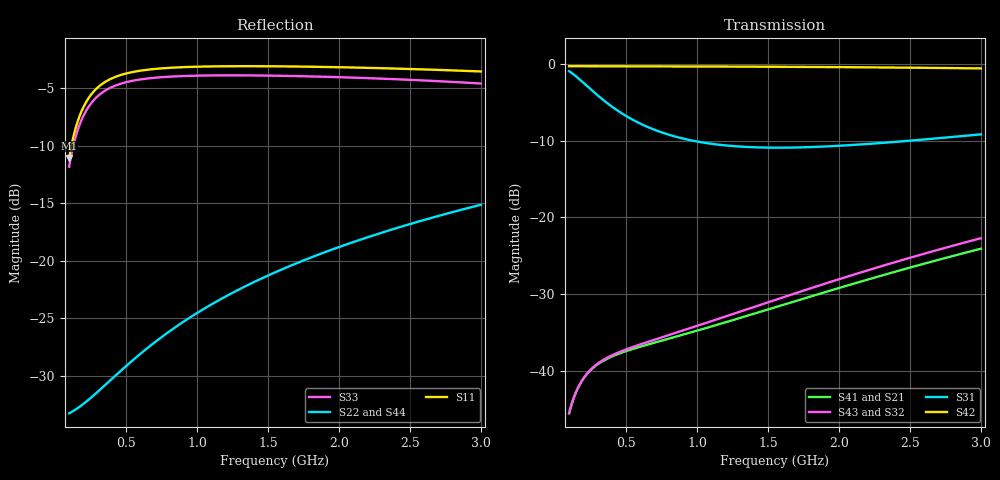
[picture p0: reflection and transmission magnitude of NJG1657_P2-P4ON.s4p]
! NJG1657MD7(1bit control high power DPDT switch) S-parameter
! VDD=2.85V, VCTL(H)=2.6V, VCTL(L)=0V
! P2-P4 ON mode
! Port1...P1, Port2...P2, Port3...P3, Port4...P4
# hz S ma R 50
! 4 Port Network Data from SP1.SP block
! freq  magS11  angS11  magS12  angS12  magS13  angS13  magS14  angS14
!  magS21  angS21  magS22  angS22  magS23  angS23  magS24  angS24
!  magS31  angS31  magS32  angS32  magS33  angS33  magS34  angS34
!  magS41  angS41  magS42  angS42  magS43  angS43  magS44  angS44
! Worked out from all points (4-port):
!   291 points, 100 MHz to 3 GHz, reference 50 ohm
!   strongest paths, dB at 100 MHz, 820 MHz, 1.55 GHz, 2.28 GHz, 3 GHz:
!     S42: -0.2, -0.3, -0.3, -0.4, -0.5
!     S31: -0.9, -9.3, -10.9, -10.3, -9.1
!     S43: -45.6, -35.3, -30.8, -26.5, -22.7
!     S32: -45.6, -35.3, -30.8, -26.5, -22.7
!     S41: -45.6, -35.7, -31.7, -27.7, -24.1
!     S21: -45.6, -35.8, -31.7, -27.7, -24.0
!   lowest |S11| = -11.1 dB at 100 MHz (marker M1), VSWR 1.77, Z = 36.3 - j20.7 ohm
!   |S11| at or under -10 dB: start of sweep to 116.5 MHz
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1e8  0.2791 -110.0  0.005241 66.2  0.9018 -17.0  0.005258 66.2
     0.005241 66.2  0.02173 -15.7  0.005264 67.1  0.9724 -1.3
     0.9018 -17.0  0.005264 67.1  0.256 -109.7  0.005272 67.0
     0.005258 66.2  0.9724 -1.3  0.005272 67.0  0.02178 -15.3
1.7e8  0.4185 -125.0  0.007918 59.8  0.8026 -25.7  0.007943 59.7
       0.007918 59.8  0.02311 -25.6  0.007969 61.2  0.9721 -2.3
       0.8026 -25.7  0.007969 61.2  0.3838 -125.0  0.007981 61.1
       0.007943 59.7  0.9721 -2.3  0.007981 61.1  0.02305 -25.2
2.8e8  0.5488 -141.3  0.01058 52.8  0.6515 -33.7  0.01061 52.7
       0.01058 52.8  0.02623 -38.9  0.0107 55.1  0.9717 -3.7
       0.6515 -33.7  0.0107 55.1  0.5031 -141.4  0.01072 54.9
       0.01061 52.7  0.9717 -3.7  0.01072 54.9  0.02594 -38.5
4.6e8  0.6394 -156.9  0.01295 49.5  0.4857 -37.0  0.01299 49.4
       0.01295 49.5  0.03309 -54.9  0.01326 53.1  0.9711 -6.1
       0.4857 -37.0  0.01326 53.1  0.586 -157.2  0.01328 52.8
       0.01299 49.4  0.9711 -6.1  0.01328 52.8  0.03232 -55.0
7.1e8  0.681 -168.9  0.01525 52.3  0.3709 -33.7  0.0153 52.1
       0.01525 52.3  0.04455 -69.5  0.01597 57.2  0.97 -9.4
       0.3709 -33.7  0.01597 57.2  0.6236 -169.4  0.01599 56.7
       0.0153 52.1  0.97 -9.4  0.01599 56.7  0.0431 -70.5
1.51e9  0.6989 172.2  0.02519 67.7  0.2857 -15.6  0.02521 67.3
        0.02519 67.7  0.08672 -94.2  0.02806 73.7  0.9642 -20.0
        0.2857 -15.6  0.02806 73.7  0.6365 170.8  0.0281 72.6
        0.02521 67.3  0.9642 -20.0  0.0281 72.6  0.08323 -98.3
3e9  0.6633 150.8  0.06303 72.7  0.3489 -3.7  0.06247 71.6
     0.06303 72.7  0.175 -122.1  0.07325 78.2  0.9403 -40.1
     0.3489 -3.7  0.07325 78.2  0.5881 147.5  0.07318 75.9
     0.06247 71.6  0.9403 -40.1  0.07318 75.9  0.1688 -131.0
